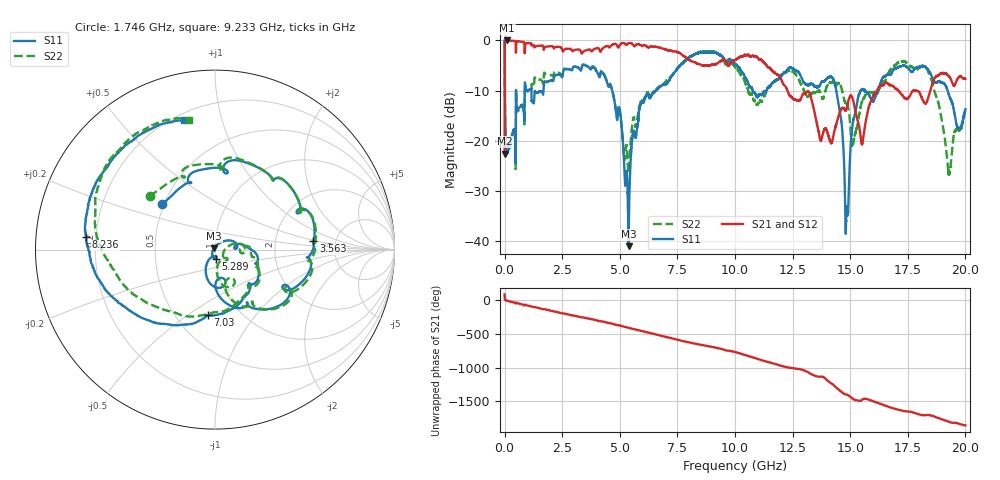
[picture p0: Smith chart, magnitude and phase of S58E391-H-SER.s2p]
!{S58E391}
!Johanson Technology Inc.
!www.johansontechnology.com
!Test Board Conditions:
!Substrate Type  RO4350B
!Substrate Thickness  60 mil
!Substrate Dk  3.66
!TL Type: GCPW
!TL Trace Width  115 mil
!TL Gap  52 mil
!Electrode orientation  Horizontal
!DUT TOPOLOGY	SERIES
!Mounting Pad LxW  55x428 mil
! Created Wed Apr 14 11:46:54 2021
# mhz S ma R 50
! 2 Port Network Data from SP1.SP block
! freq  magS11  angS11  magS21  angS21  magS12  angS12  magS22  angS22
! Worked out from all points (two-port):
!   20001 points, 300 kHz to 20 GHz, reference 50 ohm
!   highest |S21| = -0.03 dB at 113.3 MHz (marker M1); lowest = -22.5 dB at 300 kHz (marker M2)
!   |S21| within 3 dB of the highest: 4.053 MHz to 7.734 GHz (7.73 GHz wide, 200 % of centre); 10.38 GHz to 10.62 GHz (232.7 MHz wide, 2.22 % of centre)
!   lowest |S11| = -41.0 dB at 5.382 GHz (marker M3), VSWR 1.02, Z = 49.5 + j0.73 ohm
!   |S11| at or under -10 dB: 4.672 GHz to 6.562 GHz (1.89 GHz wide, 33.6 % of centre); 14.39 GHz to 15.45 GHz (1.058 GHz wide, 7.09 % of centre); 19.23 GHz to end of sweep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
!   |S22| runs from -26.8 to -0.1 dB; largest |S21 - S12| = 0.012
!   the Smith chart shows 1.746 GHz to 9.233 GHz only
!   S11 on the Smith chart (normalised r, x): 1.746 GHz: 0.49, +0.29; 3.563 GHz: 3.38, +0.46; 5.289 GHz: 1.01, -0.10; 7.03 GHz: 0.71, -0.60; 8.236 GHz: 0.16, +0.05; 9.233 GHz: 0.24, +0.76
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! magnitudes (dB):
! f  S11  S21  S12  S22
! 300 kHz  0.0  -22.5  -22.5  -0.1
! 113.3 MHz  -22.4  0.0  0.0  -22.4
! 1.746 GHz  -8.2  -1.4  -1.4  -6.5
! 3.334 GHz  -5.7  -2.5  -2.5  -5.7
! 3.563 GHz  -5.2  -2.0  -2.0  -5.1
! 4.659 GHz  -9.8  -0.9  -0.9  -9.7
! 5.289 GHz  -26.0  -0.9  -0.9  -20.9
! 5.382 GHz  -41.0  -0.6  -0.6  -26.0
! 5.919 GHz  -12.5  -1.0  -1.0  -12.1
! 6.667 GHz  -9.4  -1.4  -1.4  -9.5
! 7.03 GHz  -8.7  -1.9  -1.9  -8.0
! 8.236 GHz  -2.8  -4.3  -4.3  -2.8
! 9.233 GHz  -2.6  -4.6  -4.7  -2.7
! 10 GHz  -4.7  -3.9  -3.9  -5.3
! 13.33 GHz  -8.6  -12.0  -12.0  -10.7
! 14.32 GHz  -8.4  -17.9  -17.9  -8.8
! 14.86 GHz  -33.7  -13.4  -13.4  -12.7
! 15.39 GHz  -10.7  -17.2  -17.3  -14.7
! 16.67 GHz  -6.8  -8.8  -8.8  -6.4
! 18.31 GHz  -5.5  -12.4  -12.3  -5.5
! 19.29 GHz  -11.0  -7.2  -7.1  -26.6
! 20 GHz  -13.7  -7.7  -7.6  -13.9
